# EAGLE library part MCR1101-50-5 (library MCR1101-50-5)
Board Mount Current Sensors High Accuracy 50A Current Sensor, 5V, Ratiometric, 1.5MHz 3dB BW, OCP, Galvanic Isolation. UL/IEC/EN60950-1 and UL1577 certified. SOIC-16 Source: Datasheet
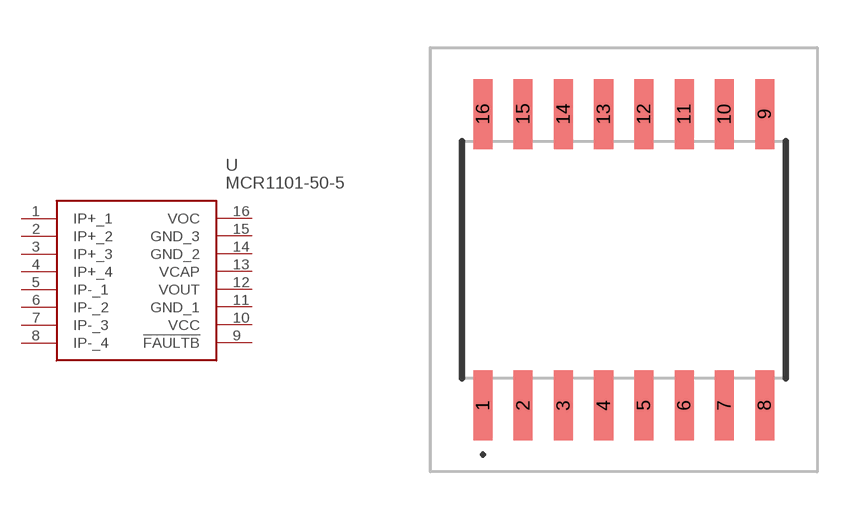
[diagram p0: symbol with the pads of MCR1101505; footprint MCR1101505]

Designator prefix U

## MCR1101-50-5 (Description: Board Mount Current Sensors High Accuracy 50A Current Sensor, 5V, Ratiometric, 1.5MHz 3dB BW, OCP, Galvanic Isolation. UL/IEC/EN60950-1 and UL1577 certified. SOIC-16; Height: 2.64mm; Manufacturer_Name: ACEINNA; Manufacturer_Part_Number: MCR1101-50-5; Mouser_Part_Number: 438-MCR1101-50-5; Mouser_Price-Stock: https://www.mouser.co.uk/ProductDetail/ACEINNA/MCR1101-50-5?qs=0lSvoLzn4L865aaRCd1YBg%3D%3D)  [MCR1101505]
1  IP+_1
2  IP+_2
3  IP+_3
4  IP+_4
5  IP-_1
6  IP-_2
7  IP-_3
8  IP-_4
9  !FAULTB
10  VCC
11  GND_1
12  VOUT
13  VCAP
14  GND_2
15  GND_3
16  VOC

## Footprint MCR1101505 (pad centres in mm)
16 Lead SOIC
smd 0.6 x 2.2: 1 -4.445,-4.6; 2 -3.175,-4.6; 3 -1.905,-4.6; 4 -0.635,-4.6; 5 0.635,-4.6; 6 1.905,-4.6; 7 3.175,-4.6; 8 4.445,-4.6; 9 4.445,4.6; 10 3.175,4.6; 11 1.905,4.6; 12 0.635,4.6; 13 -0.635,4.6; 14 -1.905,4.6; 15 -3.175,4.6; 16 -4.445,4.6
